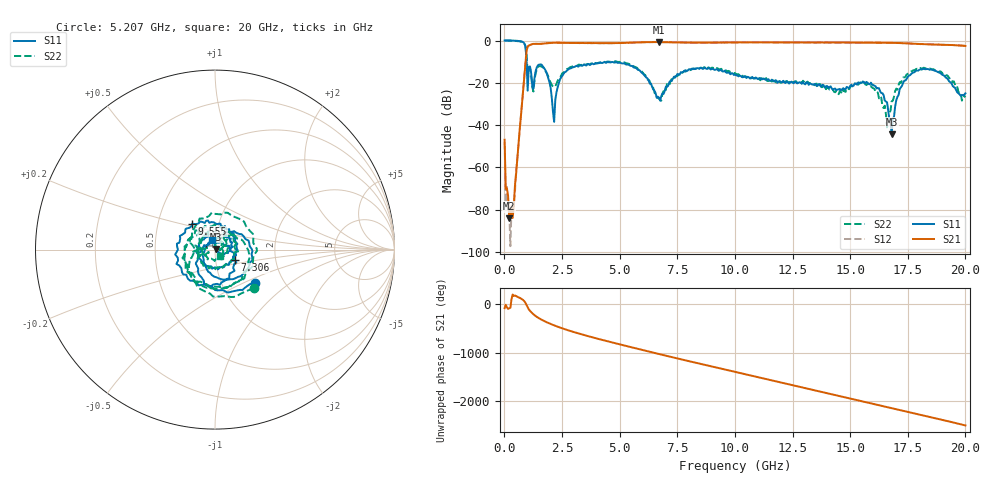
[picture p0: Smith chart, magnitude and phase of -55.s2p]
!Agilent Technologies,E8361C,US49010292,A.09.42.06
!Agilent E8361C: A.09.42.06
!Date: Wednesday, July 09, 2025 01:32:45
!Correction: S11(Full 2 Port(1,2))
!S21(Full 2 Port(1,2))
!S12(Full 2 Port(1,2))
!S22(Full 2 Port(1,2))
!S2P File: Measurements: S11, S21, S12, S22:
# Hz S  dB  R 50
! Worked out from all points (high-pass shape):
!   401 points, 10 MHz to 20 GHz, reference 50 ohm
!   highest |S21| = -0.71 dB at 6.707 GHz (marker M1); lowest = -84.1 dB at 209.9 MHz (marker M2)
!   |S21| within 3 dB of the highest: 990.3 MHz to end of sweep
!   lowest |S11| = -44.4 dB at 16.8 GHz (marker M3), VSWR 1.01, Z = 50.5 + j0.365 ohm
!   |S11| at or under -10 dB: 964.8 MHz to end of sweep
!   |S22| runs from -41.1 to 0.0 dB; largest |S21 - S12| = 0.011
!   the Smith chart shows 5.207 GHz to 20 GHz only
!   S11 on the Smith chart (normalised r, x): 5.207 GHz: 1.43, -0.58; 7.306 GHz: 1.24, -0.15; 9.555 GHz: 0.75, +0.22; 20 GHz: 0.96, +0.10
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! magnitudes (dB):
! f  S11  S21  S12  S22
! 10 MHz  0.0  -46.9  -48.1  -0.1
! 209.9 MHz  0.0  -84.1  -80.0  0.0
! 409.8 MHz  -0.1  -78.0  -78.2  -0.1
! 809.6 MHz  -0.7  -24.1  -24.1  -0.8
! 1.059 GHz  -12.5  -2.4  -2.4  -12.8
! 1.259 GHz  -22.8  -1.6  -1.6  -24.1
! 1.709 GHz  -12.9  -1.4  -1.4  -13.1
! 2.159 GHz  -38.5  -1.1  -1.1  -22.0
! 2.509 GHz  -16.8  -1.1  -1.1  -15.5
! 3.358 GHz  -12.0  -1.2  -1.2  -11.5
! 5.207 GHz  -10.8  -1.2  -1.2  -10.3
! 6.707 GHz  -27.0  -0.7  -0.7  -27.5
! 7.306 GHz  -18.1  -0.8  -0.8  -18.9
! 9.555 GHz  -14.3  -1.0  -1.0  -13.7
! 10.01 GHz  -16.2  -0.9  -0.9  -15.4
! 13.35 GHz  -20.8  -0.9  -0.9  -20.5
! 16 GHz  -21.1  -1.0  -1.1  -22.6
! 16.7 GHz  -37.3  -1.1  -1.1  -34.7
! 16.8 GHz  -44.4  -1.1  -1.1  -28.8
! 17.25 GHz  -21.3  -1.2  -1.2  -18.8
! 17.95 GHz  -14.2  -1.6  -1.6  -13.6
! 20 GHz  -25.0  -2.6  -2.5  -26.9
